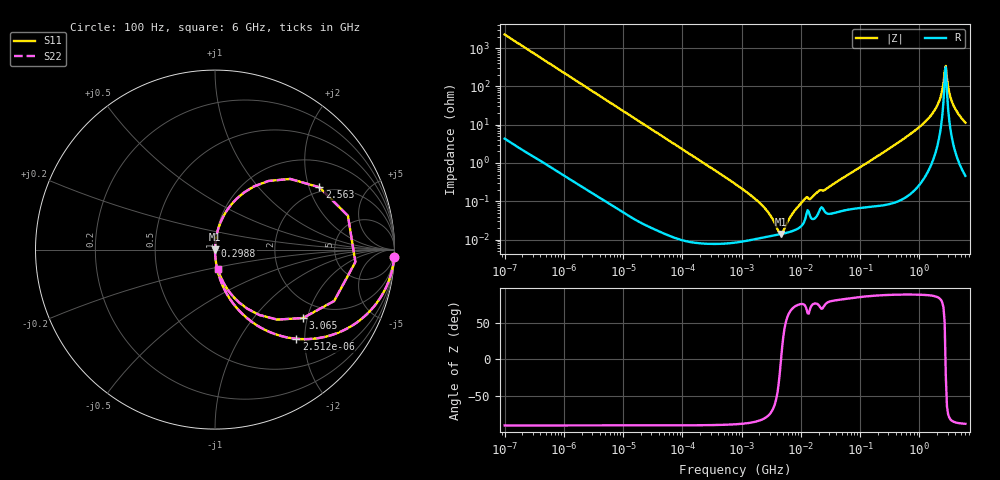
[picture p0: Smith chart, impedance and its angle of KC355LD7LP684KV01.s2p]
!Murata Part Number: KC355LD7LP684KV01
!These Parameters are Measured in Series Mode Connection
!Data Generated on Jun 19, 2026
!  o--ll--o
!Port1  Port2
!  o------o
!Operation Temp=25[degC], DC Bias Voltage=0[V]
!Freq. Start=100[Hz] Stop=6[GHz] 401[Steps]
# Hz S RI R 50
!Freq.(Hz) S11(Real) S11(Imag) S21(Real) S21(Imag) S12(Real) S12(Imag) S22(Real) S22(Imag)
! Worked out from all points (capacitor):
!   401 points, 100 Hz to 6 GHz, reference 50 ohm
!   read as one part in series: C = 699 nF near 109 Hz
!   lowest |Z| = 13.9 mohm at 4.644 MHz (marker M1)
!   series resonance near 4.631 MHz, so ESL is about 1.7 nH
!   S11 on the Smith chart (normalised r, x): 100 Hz: 1, -45; 2.512 kHz: 1.00, -1.82; 298.8 MHz: 1.00, +0.05; 2.563 GHz: 1.83, +2.35; 3.065 GHz: 1.52, -1.88; 6 GHz: 1.01, -0.23
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100  0.998 -0.0439  0.00201 0.0439  0.00201 0.0439  0.998 -0.0439
656  0.9232 -0.2653  0.0768 0.2653  0.0768 0.2653  0.9232 -0.2653
2008  0.5637 -0.4949  0.4363 0.4949  0.4363 0.4949  0.5637 -0.4949
2512  0.4526 -0.4967  0.5474 0.4967  0.5474 0.4967  0.4526 -0.4967
7358  0.0886 -0.2831  0.9114 0.2831  0.9114 0.2831  0.0886 -0.2831
40335  0.00338 -0.0566  0.9966 0.0566  0.9966 0.0566  0.00338 -0.0566
774597  9.12e-05 -0.00286  0.9999 0.00286  0.9999 0.00286  9.12e-05 -0.00286
2268635  0.000113 -0.000751  0.9999 0.000751  0.9999 0.000751  0.000113 -0.000751
4643984  0.000139 2.7e-06  0.9999 -2.7e-06  0.9999 -2.7e-06  0.000139 2.7e-06
9090158  0.000197 0.000713  0.9998 -0.000713  0.9998 -0.000713  0.000197 0.000713
1.555665e7  0.000346 0.00124  0.9997 -0.00124  0.9997 -0.00124  0.000346 0.00124
2.987521e8  0.00135 0.0228  0.9986 -0.0228  0.9986 -0.0228  0.00135 0.0228
3.124326e8  0.00141 0.0239  0.9986 -0.0239  0.9986 -0.0239  0.00141 0.0239
1.000774e9  0.0101 0.0857  0.9899 -0.0857  0.9899 -0.0857  0.0101 0.0857
1.791126e9  0.0627 0.2126  0.9373 -0.2126  0.9373 -0.2126  0.0627 0.2126
2.142435e9  0.1607 0.3175  0.8393 -0.3175  0.8393 -0.3175  0.1607 0.3175
2.562649e9  0.5816 0.3472  0.4184 -0.3472  0.4184 -0.3472  0.5816 0.3472
2.802721e9  0.782 -0.0689  0.218 0.0689  0.218 0.0689  0.782 -0.0689
3.065283e9  0.4907 -0.381  0.5093 0.381  0.5093 0.381  0.4907 -0.381
3.352442e9  0.2475 -0.3644  0.7525 0.3644  0.7525 0.3644  0.2475 -0.3644
3.8344e9  0.1044 -0.2652  0.8956 0.2652  0.8956 0.2652  0.1044 -0.2652
6e9  0.017 -0.1104  0.983 0.1104  0.983 0.1104  0.017 -0.1104
